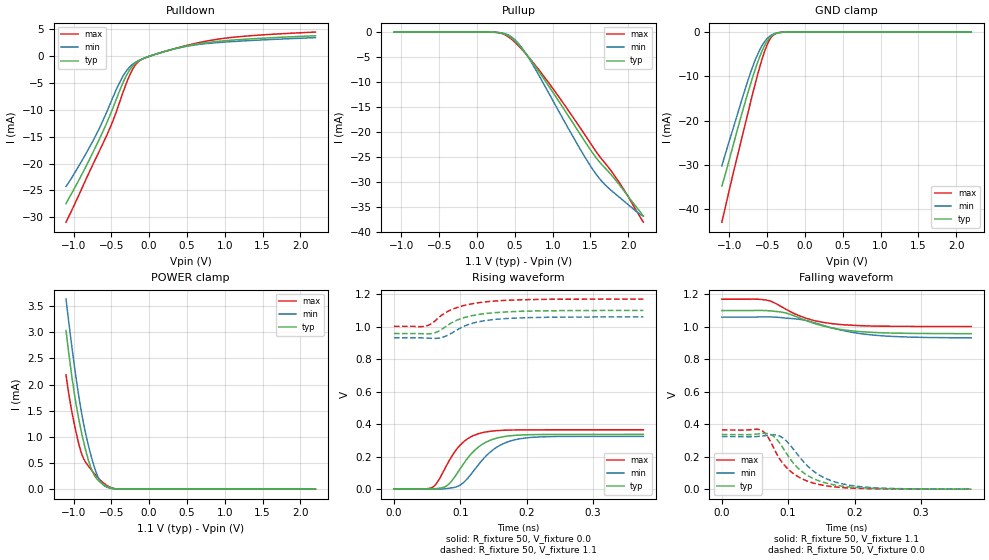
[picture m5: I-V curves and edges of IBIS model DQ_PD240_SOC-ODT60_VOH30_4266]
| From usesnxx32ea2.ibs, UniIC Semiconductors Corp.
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| DQ_PD240_SOC-ODT60_VOH30_4266
| (240 Ohm Pulldown, 60 Ohm System ODT Setting, VOH=VDDQ/3.0, 3200-4266Mbps)
[Model]   DQ_PD240_SOC-ODT60_VOH30_4266
Model_type   I/O
Vinl = 123.333mV
Vinh = 243.333mV
Vmeas = 183.333mV
Vref = 0.0mV
Cref = 0.0pF
Rref = 60.000Ohm
|   typ   min   max
|C_comp   0.834pF   0.784pF   0.884pF
C_comp_pullup   0.4170pF   0.3920pF   0.4420pF
C_comp_pulldown   0.4170pF   0.3920pF   0.4420pF
| Note: C_comp changes when the ODT circuit is enabled.
[Model Spec]
| Input threshold voltage corners
Vinl   0.1233V   0.1167V   0.1350V
Vinh   0.2433V   0.2367V   0.2550V
| Measurement voltage corners
Vmeas   0.1833V   0.1767V   0.1950V
| Timing spec test load voltage corners
Vref   0.0000V   0.0000V   0.0000V
| Dynamic Overshoot Parameters from LPDDR4 Specification
D_overshoot_ampl_h   0.30   NA   NA
D_overshoot_ampl_l   0.30   NA   NA
D_overshoot_area_h   0.1n   NA   NA
D_overshoot_area_l   0.1n   NA   NA
[Voltage Range]   1.1000V   1.0600V   1.1700V
[Pullup Reference]   1.1000V   1.0600V   1.1700V
| Junction Temperature (Ambient temp is 35C typ 95C min -40C max)
[Temperature Range]   50.0   110.0   -40.0
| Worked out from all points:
|   slope of the pulldown table from 0 to 0.165 V, typ, clamps not added: 223 ohm
|   slope of the pullup table from 0 to 0.165 V, typ, clamps not added: 19.4 kohm
|   GND clamp passes 1 mA (typ) near -0.45 V on its own axis
|   POWER clamp passes 1 mA (typ) near -0.88 V on its own axis
|   rising waveform, R_fixture 50, V_fixture 0.0: 20-80 % time 40.6ps typ, 44.8ps min, 35.3ps max; typ from 0.001 V to 0.337 V
|   falling waveform, R_fixture 50, V_fixture 1.1: 20-80 % time 68.5ps typ, 78.1ps min, 58.1ps max; typ from 1.1 V to 0.958 V
|   rising waveform, R_fixture 50, V_fixture 1.1: 20-80 % time 49.4ps typ, 47.5ps min, 50.5ps max; typ from 0.958 V to 1.1 V
|   falling waveform, R_fixture 50, V_fixture 0.0: 20-80 % time 47.1ps typ, 51.6ps min, 43.1ps max; typ from 0.337 V to 0.001 V
[Pulldown]
|   Voltage   I(typ)   I(min)   I(max)
-1.1V     -27.48mA   -24.26mA   -30.94mA
-921.8mV  -22.88mA   -20.24mA   -25.63mA
-717.2mV  -17.17mA   -15.08mA   -19.39mA
-502.7mV  -10.47mA   -8.452mA   -12.86mA
-344.3mV  -4.883mA   -3.676mA   -6.675mA
-228.8mV  -1.996mA   -1.62mA    -2.701mA
-182.6mV  -1.317mA   -1.143mA   -1.644mA
-123.2mV  -746.2uA   -693.6uA   -809.7uA
375.1mV   1.526mA    1.498mA    1.571mA
843.7mV   2.68mA     2.467mA    3.039mA
1.355V    3.244mA    2.938mA    3.836mA
2.2V      3.814mA    3.471mA    4.502mA
[GND Clamp]
|   Voltage   I(typ)   I(min)   I(max)
-1.1V     -34.74mA   -30.21mA   -42.91mA
-1.05V    -31.86mA   -27.33mA   -39.27mA
-935mV    -24.6mA    -20.89mA   -30.85mA
-793.1mV  -15.92mA   -12.96mA   -20.95mA
-664.4mV  -8.736mA   -6.578mA   -12.07mA
-591.8mV  -5.255mA   -3.789mA   -7.493mA
-522.5mV  -2.665mA   -1.905mA   -3.811mA
-466.4mV  -1.296mA   -944.3uA   -1.691mA
-416.9mV  -596.8uA   -441.6uA   -665.1uA
-354.2mV  -178.8uA   -135uA     -160uA
-255.2mV  -14.81uA   -13.09uA   -8.787uA
2.2V      0A         0A         0A
[Pullup]
|   Voltage   I(typ)   I(min)   I(max)
-1.1V     4.184uA    6.447uA    1.886uA
229.9mV   -30.26uA   -30.87uA   -31.04uA
332.2mV   -215uA     -179.9uA   -295.3uA
434.5mV   -925.5uA   -758.7uA   -1.171mA
546.7mV   -2.488mA   -2.279mA   -2.716mA
678.7mV   -4.971mA   -5.087mA   -4.942mA
1.088V    -14.01mA   -16.05mA   -13.11mA
1.388V    -21.03mA   -24.07mA   -19.73mA
1.576V    -25.2mA    -28.5mA    -23.98mA
1.688V    -27.16mA   -30.52mA   -26.18mA
1.887V    -30.68mA   -33.15mA   -30.26mA
2.2V      -36.89mA   -36.87mA   -38.1mA
[POWER Clamp]
|   Voltage   I(typ)   I(min)   I(max)
-1.1V     3.033mA    3.633mA    2.184mA
-1.044V   2.381mA    2.967mA    1.653mA
-977.9mV  1.723mA    2.241mA    1.161mA
-908.6mV  1.177mA    1.582mA    748.3uA
-852.5mV  818.2uA    1.148mA    543.5uA
-776.6mV  434.2uA    683.3uA    390.2uA
-710.6mV  232.2uA    359.1uA    273.1uA
-654.5mV  142.6uA    170.5uA    185.9uA
-598.4mV  83.66uA    71.98uA    113uA
-489.5mV  17.78uA    10.87uA    22.46uA
-367.4mV  1.186uA    875nA      943.4nA
2.2V      0A         0A         0A
[Ramp]
|   typ   min   max
| 20% - 80%
dV/dt_r   201.65m/40.56p   194.40m/44.80p   218.77m/35.31p
dV/dt_f   85.16m/68.48p   76.64m/78.18p   100.79m/58.27p
| 25% - 75%
|dV/dt_r   168.05m/32.33p   162.00m/35.68p   182.31m/28.11p
|dV/dt_f   70.97m/54.49p   63.86m/61.99p   83.99m/46.29p
R_load = 50
[Rising Waveform]
R_fixture = 50
V_fixture = 0.0
|   Time   V(typ)   V(min)   V(max)
0s        757uV      671.7uV    544.7uV
57ps      502.7uV    -132.1uV   8.968mV
65ps      3.285mV    -327.9uV   39.69mV
77ps      14.32mV    2.387mV    127.4mV
90ps      65.91mV    9.777mV    219.9mV
104ps     151.2mV    37.02mV    287.5mV
134ps     277.7mV    182.5mV    348.4mV
160ps     318.7mV    269.9mV    361.3mV
194ps     333.6mV    312.5mV    364.6mV
376ps     336.8mV    324.7mV    365.2mV
[Falling Waveform]
R_fixture   = 50
V_fixture   = 1.1
V_fixture_min = 1.06
V_fixture_max = 1.17
|   Time   V(typ)   V(min)   V(max)
0s        1.1V       1.06V      1.17V
67ps      1.1V       1.061V     1.165V
74ps      1.098V     1.061V     1.158V
94ps      1.088V     1.055V     1.114V
126ps     1.041V     1.04V      1.054V
144ps     1.015V     1.02V      1.034V
169ps     990.7mV    990.1mV    1.018V
203ps     972.4mV    961.7mV    1.008V
243ps     963.2mV    944.4mV    1.004V
376ps     958.1mV    932.3mV    1.002V
[Rising Waveform]
R_fixture   = 50
V_fixture   = 1.1
V_fixture_min = 1.06
V_fixture_max = 1.17
|   Time   V(typ)   V(min)   V(max)
0s        957.9mV    931.6mV    1.002V
45ps      956.1mV    930.6mV    1.001V
57ps      957.6mV    928mV      1.02V
70ps      978.3mV    931.1mV    1.064V
85ps      1.019V     955.5mV    1.102V
102ps     1.051V     995.5mV    1.126V
119ps     1.069V     1.022V     1.142V
140ps     1.082V     1.039V     1.154V
203ps     1.096V     1.056V     1.167V
376ps     1.1V       1.06V      1.17V
[Falling Waveform]
R_fixture = 50
V_fixture = 0.0
|   Time   V(typ)   V(min)   V(max)
0s        336.9mV    324.8mV    365.2mV
56ps      341.6mV    325.6mV    368.1mV
74ps      336.5mV    334.8mV    288.7mV
87ps      285.9mV    327.7mV    188mV
101ps     198.4mV    281.2mV    119.6mV
119ps     114.9mV    189.1mV    68.42mV
143ps     56.99mV    97.18mV    32.73mV
171ps     25.76mV    44.46mV    14.19mV
208ps     9.432mV    16.47mV    4.912mV
376ps     911.3uV    965.7uV    603.5uV
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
